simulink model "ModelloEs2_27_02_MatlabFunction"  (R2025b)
settings: Solver=FixedStepAuto  StartTime=0.0  StopTime=Tsim  FixedStep=Tc  RelTol=1e-3
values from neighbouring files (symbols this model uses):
  a = 25    [ScriptEs2_27_02.m]    (also in ScriptEs2_26_02.m = 5)
  x0 = 2    [ScriptEs2_27_02.m]    (also in ScriptEs2_26_02.m = 1)
  y0 = -1    [ScriptEs2_27_02.m]    (also in ScriptEs2_26_02.m)
  y0punto = 1    [ScriptEs2_27_02.m]

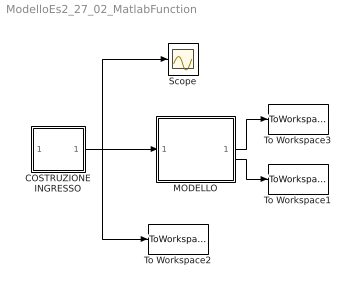
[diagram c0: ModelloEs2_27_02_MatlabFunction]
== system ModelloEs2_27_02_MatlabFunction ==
  COSTRUZIONE INGRESSO : Subsystem
  MODELLO : Subsystem
  Scope : Scope
  To Workspace1 : ToWorkspace  VariableName=y  SaveFormat=Timeseries  SampleTime=-1
  To Workspace2 : ToWorkspace  VariableName=u  SaveFormat=Timeseries  SampleTime=-1
  To Workspace3 : ToWorkspace  VariableName=x  SaveFormat=Timeseries  SampleTime=-1
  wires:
  COSTRUZIONE INGRESSO/1(u(t)) -> To Workspace2/1, Scope/1, MODELLO/1(u(t))
  MODELLO/2(y(t)) -> To Workspace1/1
  MODELLO/1(x(t)) -> To Workspace3/1

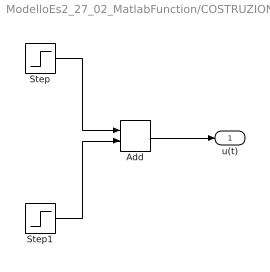
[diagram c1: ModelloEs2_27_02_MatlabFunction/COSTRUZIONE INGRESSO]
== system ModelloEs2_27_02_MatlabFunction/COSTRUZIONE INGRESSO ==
  Add : Sum
  Step : Step  Time=3  Before=2  After=4  SampleTime=0
  Step1 : Step  Time=6  After=0.5  SampleTime=0
  u(t) : Outport
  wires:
  Step/1 -> Add/1
  Step1/1 -> Add/2
  Add/1 -> u(t)/1

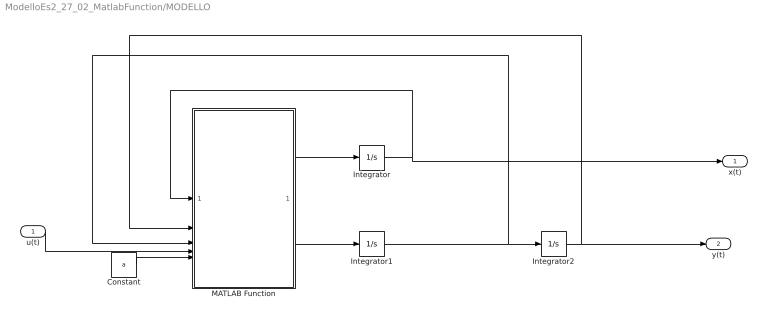
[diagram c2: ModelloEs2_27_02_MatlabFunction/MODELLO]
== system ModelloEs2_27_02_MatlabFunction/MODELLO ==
  u(t) : Inport
  Constant : Constant  Value=a
  Integrator : Integrator  InitialCondition=x0
  Integrator1 : Integrator  InitialCondition=y0punto
  Integrator2 : Integrator  InitialCondition=y0
  MATLAB Function : MATLAB Function  TreatAsAtomicUnit=on
  x(t) : Outport
  y(t) : Outport  Port=2
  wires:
  Integrator1/1 -> Integrator2/1, MATLAB Function/3(ydot)
  MATLAB Function/1(xdot) -> Integrator/1
  u(t)/1 -> MATLAB Function/4(u)
  Constant/1 -> MATLAB Function/5(a)
  MATLAB Function/2(yddot) -> Integrator1/1
  Integrator/1 -> x(t)/1, MATLAB Function/1(x)
  Integrator2/1 -> y(t)/1, MATLAB Function/2(y)

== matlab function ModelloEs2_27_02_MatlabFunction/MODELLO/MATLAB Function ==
function [xdot,yddot] = fcn(x,y,ydot,u,a)

xdot=-2*x/(1+abs(x))+2*cos(x+y)+2*sin(y);
yddot=-0.5*a*sin(y)+x/(1+abs(x))+0.5*u;
